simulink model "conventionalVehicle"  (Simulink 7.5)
settings: Solver=ode45  StartTime=0.0  StopTime=Tfinal  RelTol=1e-3
InitFcn:
  | t_Start=tic;
StopFcn:
  | t_elapsed=toc(t_Start);
  | fuel_cons=(1000*(fueltank_simple1_std(end,1)/fueltank_simple1_std(end,3)))/(chassis_simple4_std(end,2)/100000);
  | 
  | disp(' ')
  | disp(['Time Elapsed: ' num2str(round(100*t_elapsed)/100) 's'])
  | disp(['Fuel Consumption: ' num2str(round(1000*fuel_cons)/1000) 'L/100km'])
undefined symbols (not defined in the file or in its folder): computed_mass, DC, levelinit
libraries: simulink x10, simulink_extras x2
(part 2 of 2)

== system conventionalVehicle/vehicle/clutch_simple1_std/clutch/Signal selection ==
  torque_out : Inport  OutDataType=sfix(16)  OutScaling=2^0
  torque_in : Inport  Port=2  OutDataType=sfix(16)  OutScaling=2^0
  inertia : Inport  Port=3  OutDataType=sfix(16)  OutScaling=2^0
  speed1 : Inport  Port=4  OutDataType=sfix(16)  OutScaling=2^0
  speed_fb : Inport  Port=5  OutDataType=sfix(16)  OutScaling=2^0
  logic : Inport  Port=6  OutDataType=sfix(16)  OutScaling=2^0
  Constant : Constant  Value=inertia  OutDataType=sfix(16)  OutScaling=2^0
  Memory2 : Memory
  Sum : Sum  OutDataType=sfix(16)  OutScaling=2^0
  Switch : Switch  Threshold=0.5
  Switch1 : Switch  Threshold=0.5
  Switch2 : Switch  Threshold=0.5
  torque : Outport  OutDataType=sfix(16)  OutScaling=2^0
  inertia_out : Outport  Port=2  OutDataType=sfix(16)  OutScaling=2^0
  speed : Outport  Port=3  OutDataType=sfix(16)  OutScaling=2^0
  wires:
  Sum/1 -> Switch1/3
  Constant/1 -> Switch1/1, Sum/1
  inertia/1 -> Sum/2
  speed1/1 -> Switch2/1
  speed_fb/1 -> Switch2/3
  logic/1 -> Switch1/2, Switch/2, Memory2/1
  torque_in/1 -> Switch/3
  torque_out/1 -> Switch/1
  Switch/1 -> torque/1
  Switch1/1 -> inertia_out/1
  Switch2/1 -> speed/1
  Memory2/1 -> Switch2/2

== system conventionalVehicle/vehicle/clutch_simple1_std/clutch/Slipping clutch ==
  Clutch_ctrl : Inport  OutDataType=sfix(16)  OutScaling=2^0
  torque_in : Inport  Port=2  OutDataType=sfix(16)  OutScaling=2^0
  inertia : Inport  Port=3  OutDataType=sfix(16)  OutScaling=2^0
  speed_fb : Inport  Port=4  OutDataType=sfix(16)  OutScaling=2^0
  logic : Inport  Port=5  OutDataType=sfix(16)  OutScaling=2^0
  Clutch : Subsystem
  Flywheel : Subsystem
  Scope : Scope
  torque : Outport  OutDataType=sfix(16)  OutScaling=2^0
  speed : Outport  Port=2  OutDataType=sfix(16)  OutScaling=2^0
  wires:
  torque_in/1 -> Flywheel/2(torque_in)
  Flywheel/1(speed) -> speed/1, Clutch/3(speed)
  logic/1 -> Clutch/4(logic), Flywheel/4(logic)
  speed_fb/1 -> Clutch/2(speed_fb), Flywheel/5(speed_fb)
  inertia/1 -> Flywheel/3(inertia)
  Clutch/1(torque_out) -> Flywheel/1(torque_out), torque/1, Scope/1
  Clutch_ctrl/1 -> Clutch/1(clutch_ctrl)

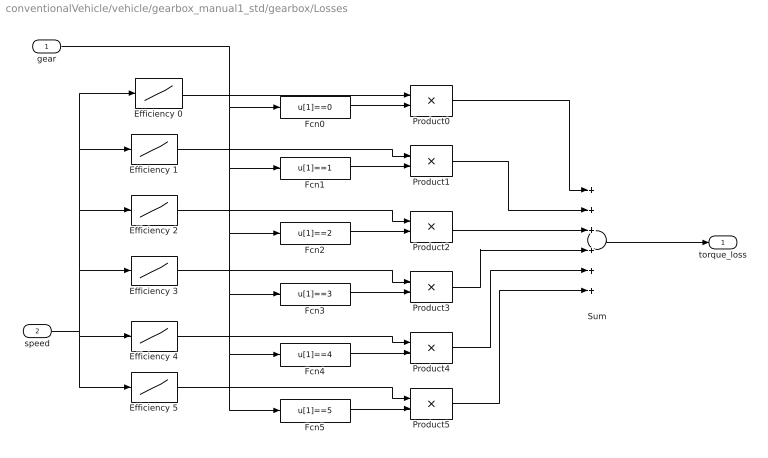
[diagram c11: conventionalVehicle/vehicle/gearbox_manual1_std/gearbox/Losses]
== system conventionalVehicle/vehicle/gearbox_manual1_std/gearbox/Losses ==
  gear : Inport  OutDataType=sfix(16)  OutScaling=2^0
  speed : Inport  Port=2  OutDataType=sfix(16)  OutScaling=2^0
  Efficiency 0 : Lookup  InputValues=gearloss_tabIp  Table=gearloss_tab0  OutDataType=sfix(16)  OutScaling=2^0
  Efficiency 1 : Lookup  InputValues=gearloss_tabIp  Table=gearloss_tab1  OutDataType=sfix(16)  OutScaling=2^0
  Efficiency 2 : Lookup  InputValues=gearloss_tabIp  Table=gearloss_tab2  OutDataType=sfix(16)  OutScaling=2^0
  Efficiency 3 : Lookup  InputValues=gearloss_tabIp  Table=gearloss_tab3  OutDataType=sfix(16)  OutScaling=2^0
  Efficiency 4 : Lookup  InputValues=gearloss_tabIp  Table=gearloss_tab4  OutDataType=sfix(16)  OutScaling=2^0
  Efficiency 5 : Lookup  InputValues=gearloss_tabIp  Table=gearloss_tab5  OutDataType=sfix(16)  OutScaling=2^0
  Fcn0 : Fcn  Expr=u[1]==0
  Fcn1 : Fcn  Expr=u[1]==1
  Fcn2 : Fcn  Expr=u[1]==2
  Fcn3 : Fcn  Expr=u[1]==3
  Fcn4 : Fcn  Expr=u[1]==4
  Fcn5 : Fcn  Expr=u[1]==5
  Product{0..5} (6 alike) : Product  OutDataType=sfix(16)  OutScaling=2^0
  Sum : Sum  Inputs=++++++  OutDataType=sfix(16)  OutScaling=2^0
  torque_loss : Outport  OutDataType=sfix(16)  OutScaling=2^0
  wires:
  Efficiency 5/1 -> Product5/1
  Efficiency 4/1 -> Product4/1
  Efficiency 3/1 -> Product3/1
  Efficiency 2/1 -> Product2/1
  Efficiency 1/1 -> Product1/1
  Efficiency 0/1 -> Product0/1
  speed/1 -> Efficiency 0/1, Efficiency 1/1, Efficiency 2/1, Efficiency 3/1, Efficiency 4/1, Efficiency 5/1
  gear/1 -> Fcn4/1, Fcn5/1, Fcn3/1, Fcn2/1, Fcn1/1, Fcn0/1
  Product0/1 -> Sum/1
  Product1/1 -> Sum/2
  Product2/1 -> Sum/3
  Product3/1 -> Sum/4
  Product4/1 -> Sum/5
  Product5/1 -> Sum/6
  Fcn5/1 -> Product5/2
  Fcn4/1 -> Product4/2
  Fcn3/1 -> Product3/2
  Fcn2/1 -> Product2/2
  Fcn1/1 -> Product1/2
  Sum/1 -> torque_loss/1
  Fcn0/1 -> Product0/2

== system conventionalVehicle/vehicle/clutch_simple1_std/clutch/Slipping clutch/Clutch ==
  clutch_ctrl : Inport  OutDataType=sfix(16)  OutScaling=2^0
  speed_fb : Inport  Port=2  OutDataType=sfix(16)  OutScaling=2^0
  speed : Inport  Port=3  OutDataType=sfix(16)  OutScaling=2^0
  logic : Inport  Port=4  OutDataType=sfix(16)  OutScaling=2^0
  Gain : Gain  Gain=max_torque  ParameterDataType=sfix(16)  ParameterScaling=2^0  OutDataType=sfix(16)  OutScaling=2^0
  Product : Product  OutDataType=sfix(16)  OutScaling=2^0
  Product1 : Product  OutDataType=sfix(16)  OutScaling=2^0
  Sign : Signum
  Sum : Sum  Inputs=-+  OutDataType=sfix(16)  OutScaling=2^0
  torque_out : Outport  OutDataType=sfix(16)  OutScaling=2^0
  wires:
  Product/1 -> Gain/1
  Product1/1 -> Sign/1
  logic/1 -> Product1/2
  Sum/1 -> Product1/1
  speed/1 -> Sum/2
  speed_fb/1 -> Sum/1
  clutch_ctrl/1 -> Product/1
  Sign/1 -> Product/2
  Gain/1 -> torque_out/1

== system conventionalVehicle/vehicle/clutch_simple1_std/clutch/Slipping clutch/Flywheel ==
  torque_out : Inport  OutDataType=sfix(16)  OutScaling=2^0
  torque_in : Inport  Port=2  OutDataType=sfix(16)  OutScaling=2^0
  inertia : Inport  Port=3  OutDataType=sfix(16)  OutScaling=2^0
  logic : Inport  Port=4  OutDataType=sfix(16)  OutScaling=2^0
  speed_fb : Inport  Port=5  OutDataType=sfix(16)  OutScaling=2^0
  Integrator : Integrator  ExternalReset=rising  InitialConditionSource=external  InitialCondition=0.001  LowerSaturationLimit=-eps
  Memory2 : Memory
  Product : Product  Inputs=*/  OutDataType=sfix(16)  OutScaling=2^0
  Sum : Sum  Inputs=-+  OutDataType=sfix(16)  OutScaling=2^0
  speed : Outport  OutDataType=sfix(16)  OutScaling=2^0
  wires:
  Integrator/1 -> speed/1
  torque_in/1 -> Sum/2
  inertia/1 -> Product/2
  Product/1 -> Integrator/1
  speed_fb/1 -> Integrator/3
  logic/1 -> Memory2/1
  Sum/1 -> Product/1
  torque_out/1 -> Sum/1
  Memory2/1 -> Integrator/2
